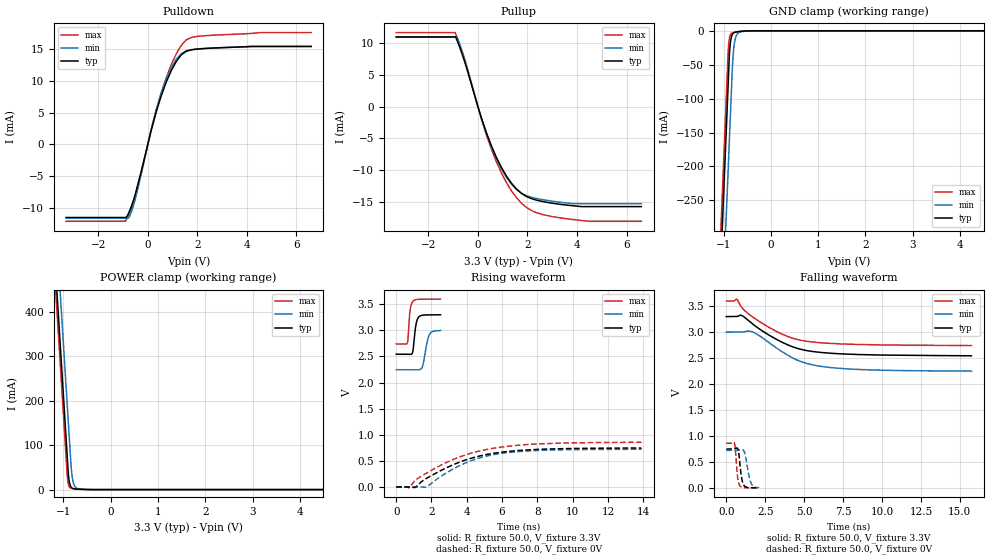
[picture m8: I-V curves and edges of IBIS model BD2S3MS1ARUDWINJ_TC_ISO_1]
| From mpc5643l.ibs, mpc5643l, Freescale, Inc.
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| *** New cell (Generated with 5.14beta1 (Sep 20 2010 13:23:23))
[Model]   BD2S3MS1ARUDWINJ_TC_ISO_1
Model_type I/O
Polarity   Non-Inverting
Enable   Active-Low
| CAP_THRESHOLD on pad pad is "CMOS" :
| Rising=10.0% of VDDE1   Falling=90.0% of VDDE1
| C_comp min and max val. don't necessarily correlate with the min and max pvt
| but are the smallest and greatest pad capacitance found.
| var   typ   min   max
C_comp   1.91462pF  1.76636pF  2.10960pF
Vinl = 1.05V | Dummy value overriden by next lines
Vinh = 2.34V | Dummy value overriden by next lines
Vmeas = 1.65V   | Reference voltage for timing measurements
Cref  = 25.0pF   | Timing specification test load capacitance value
Rref  = 1.0MOhm   | Timing specification test load resistance value
Vref  = 1.65V   | Timing specification test load voltage
[Model Spec]
| TIME_THRESHOLD on pin ipp_ind is "CORE" :
| Rising=40.0% of VDD   Falling=60.0% of VDD
Vinl 1.30950V 1.19650V 1.40650V
Vinh 1.89650V 1.72150V 2.04550V
| variable   typ   min   max
[Temperature Range] 25.0 150.0 -40.0
| variable   typ   min   max
[Voltage Range] 3.3V 3.0V 3.6V
| variable   typ   min   max
[POWER Clamp Reference] 3.3V 3.0V 3.6V
| variable   typ   min   max
[GND Clamp Reference] 0V 0V 0V
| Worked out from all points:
|   slope of the pulldown table from 0 to 0.495 V, typ, clamps not added: 70.3 ohm
|   slope of the pullup table from 0 to 0.495 V, typ, clamps not added: 86.8 ohm
|   GND clamp passes 1 mA (typ) near -0.66 V on its own axis
|   POWER clamp passes 1 mA (typ) near -0.67 V on its own axis
|   rising waveform, R_fixture 50.0, V_fixture 3.3V: 20-80 % time 161ps typ, 252ps min, 125ps max; typ from 2.54 V to 3.3 V
|   falling waveform, R_fixture 50.0, V_fixture 3.3V: 20-80 % time 2.75ns typ, 2.64ns min, 2.84ns max; typ from 3.3 V to 2.54 V
|   rising waveform, R_fixture 50.0, V_fixture 0V: 20-80 % time 3.15ns typ, 2.69ns min, 3.43ns max; typ from 0 V to 0.748 V
|   falling waveform, R_fixture 50.0, V_fixture 0V: 20-80 % time 178ps typ, 269ps min, 142ps max; typ from 0.748 V to 0 V
[POWER Clamp]
-3.3V     4.126A     4.242A     4.083A
-1.21V    573.2mA    689.5mA    530.1mA
-1.14V    454.2mA    570.5mA    411.1mA
-1.07V    335.2mA    451.5mA    292.1mA
-1V       216.2mA    332.5mA    173.1mA
-910mV    63.16mA    179.5mA    23.78mA
-880mV    22.46mA    128.5mA    7.535mA
-840mV    6.363mA    60.49mA    3.143mA
-810mV    3.226mA    27.5mA     2.363mA
-770mV    1.895mA    10.15mA    1.875mA
-620mV    704.1uA    944.2uA    740.5uA
6.6V      0A         0A         0A
[GND Clamp]
-3.3V     -4.155A    -4.281A    -4.106A
-1.08V    -381.2mA   -507mA     -332.5mA
-910mV    -92.2mA    -218mA     -43.47mA
-890mV    -58.2mA    -184mA     -18.35mA
-870mV    -28.89mA   -150mA     -8.87mA
-850mV    -14.77mA   -116mA     -5.18mA
-810mV    -4.979mA   -50.04mA   -2.894mA
-780mV    -2.923mA   -23.23mA   -2.281mA
-740mV    -1.887mA   -8.971mA   -1.729mA
-680mV    -1.179mA   -2.825mA   -1.072mA
-560mV    -377.4uA   -728uA     -262.1uA
6.6V      11.35nA    2.809uA    94.3pA
| variable   typ   min   max
[Pullup Reference] 3.3V 3.0V 3.6V
| variable   typ   min   max
[Pulldown Reference] 0V 0V 0V
[Pullup]
-3.3V     11.03mA    10.98mA    11.72mA
-920mV    11.03mA    10.98mA    11.72mA
-840mV    10.45mA    10.98mA    10.94mA
-710mV    9.112mA    9.542mA    9.573mA
-470mV    6.281mA    6.567mA    6.637mA
140mV     -1.782mA   -1.838mA   -1.918mA
740mV     -7.979mA   -8.178mA   -8.659mA
1.35V     -12.08mA   -12.23mA   -13.28mA
1.96V     -14.21mA   -14.08mA   -15.93mA
2.57V     -14.96mA   -14.67mA   -17mA
3.78V     -15.65mA   -15.31mA   -17.82mA
6.6V      -15.8mA    -15.33mA   -18.12mA
[Pulldown]
-3.3V     -11.5mA    -11.61mA   -12.09mA
-890mV    -11.5mA    -11.61mA   -11.99mA
-740mV    -10.5mA    -11.31mA   -10.8mA
-550mV    -8.419mA   -9.215mA   -8.653mA
-270mV    -4.331mA   -4.79mA    -4.454mA
140mV     2.228mA    2.408mA    2.326mA
340mV     5.098mA    5.459mA    5.363mA
740mV     9.751mA    10.23mA    10.43mA
1.15V     13.03mA    13.37mA    14.23mA
1.55V     14.63mA    14.7mA     16.41mA
2.54V     15.11mA    15.12mA    17.13mA
6.6V      15.41mA    15.34mA    17.57mA
[Ramp]
dV/dt_r 448.50127mV/3.15223ns 433.17527mV/2.68547ns 515.1057mV/3.4347ns
dV/dt_f 453.48232mV/2.74638ns 451.76698mV/2.64256ns 515.2916mV/2.84211ns
R_load = 50.0
| Removed startup time: 0s 0s 0s  .
| Removed end time: 2.51ns.
[Rising Waveform]
R_fixture   = 50.0
V_fixture   = 3.3V
V_fixture_min = 3.0V
V_fixture_max = 3.6V
0s        2.544V     2.247V     2.741V
629ps     2.544V     2.247V     2.758V
788ps     2.54V      2.247V     3.385V
972ps     2.663V     2.247V     3.566V
1.114ns   3.099V     2.246V     3.59V
1.273ns   3.256V     2.244V     3.596V
1.501ns   3.292V     2.318V     3.598V
1.75ns    3.297V     2.771V     3.599V
1.895ns   3.298V     2.927V     3.599V
2.512ns   3.3V       2.999V     3.6V
| Removed startup time: 0s 0s 0s  .
| Removed end time: 15.741ns.
[Falling Waveform]
R_fixture   = 50.0
V_fixture   = 3.3V
V_fixture_min = 3.0V
V_fixture_max = 3.6V
0s        3.3V       3V         3.6V
450ps     3.3V       3V         3.6V
666ps     3.301V     3V         3.635V
1.056ns   3.312V     3.002V     3.453V
1.695ns   3.157V     3.005V     3.291V
3.513ns   2.815V     2.636V     2.971V
4.977ns   2.656V     2.414V     2.832V
6.276ns   2.604V     2.333V     2.79V
8.202ns   2.572V     2.285V     2.765V
15.75ns   2.544V     2.247V     2.741V
| Removed startup time: 0s 0s 0s  .
| Removed end time: 13.89ns.
[Rising Waveform]
R_fixture   = 50.0
V_fixture   = 0V
V_fixture_min = 0V
V_fixture_max = 0V
0s        13.68nV    798.4nV    13.08nV
723ps     596.5uV    -333.5nV   -17.65mV
1.062ns   -10.54mV   249uV      120.4mV
1.665ns   152.7mV    -4.334mV   253.7mV
2.757ns   351.7mV    250.1mV    453mV
3.675ns   485.7mV    421.4mV    584.6mV
4.476ns   571mV      529.5mV    667.7mV
5.376ns   636.2mV    608.8mV    733.7mV
7.926ns   717.6mV    696.9mV    821.9mV
13.9ns    747.5mV    722mV      858.5mV
| Removed startup time: 0s 0s 0s  .
| Removed end time: 2.082ns.
[Falling Waveform]
R_fixture   = 50.0
V_fixture   = 0V
V_fixture_min = 0V
V_fixture_max = 0V
0s        747.5mV    722mV      858.5mV
526ps     751.6mV    721.8mV    859.2mV
580ps     759mV      721.7mV    752.9mV
714ps     761.3mV    722mV      223.7mV
792ps     686.7mV    725mV      95.21mV
870ps     469.8mV    730.6mV    40.88mV
991ps     173.5mV    739.5mV    13.37mV
1.145ns   43.11mV    704mV      3.601mV
1.58ns    2.2mV      97.66mV    472.1uV
2.084ns   163.1uV    298.9uV    127.9uV
